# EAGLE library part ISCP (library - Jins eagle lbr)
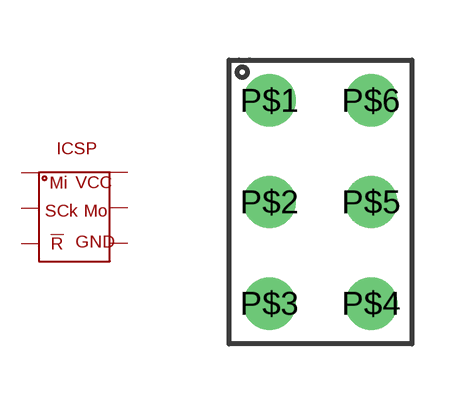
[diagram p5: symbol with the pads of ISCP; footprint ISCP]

Designator prefix -

## ISCP-6PINS  [ISCP]
P$1  P$1
P$2  P$2
P$3  P$3
P$4  P$4
P$5  P$5
P$6  P$6

## Footprint ISCP (pad centres in mm)
drill 0.8: P$1 -2.54,2.54; P$2 -2.54,0; P$3 -2.54,-2.54; P$4 0,-2.54; P$5 0,0; P$6 0,2.54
